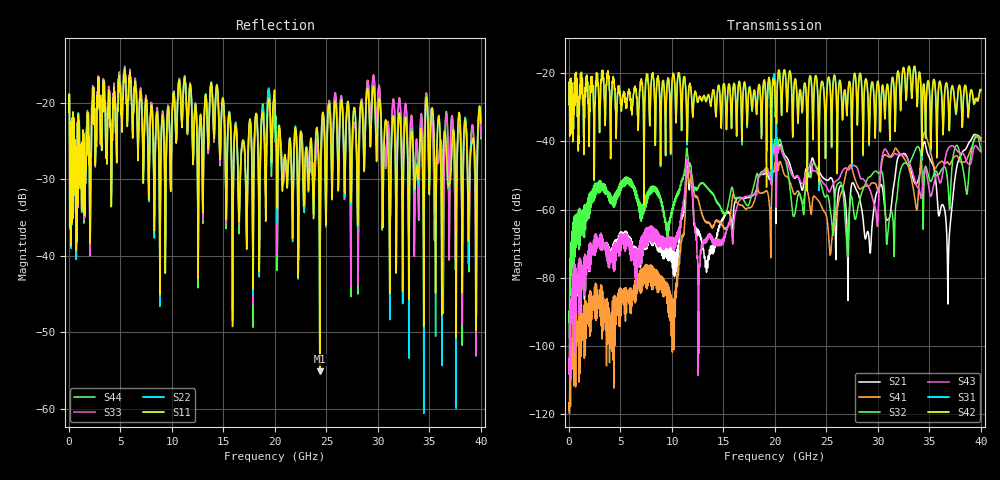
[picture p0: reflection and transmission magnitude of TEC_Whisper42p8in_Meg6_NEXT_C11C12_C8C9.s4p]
! Tyco Electronics Strada Whisper System
! NEXT_C11C12-C8C9
!! SYSTEM DESCRIPTION: Daughtercard-Connector-Backplane-Connector-Daughtercard
!! PCB DESCRIPTION: BP: 250mil, 26 lyrs, Megtron6, bottom layer route, no stub, 6-9-6mil 30" traces; DC: 150mil, 16 lyrs, Megtron6, bottom layer route, no stub, 6-9-6mil 5" traces
!! CONNECTOR DESCRIPTION: STRADA Whisper, Right Angle Receptacle to Vertical Header
!! MODEL DESCRIPTION: Tyco Electronics System 4-port S-parameter
!! MODEL STATUS: Developmental
!! MODEL GEOMETRY: Channel Model
!! MODEL FREQUENCY RANGE: DC to 40 GHz in 10 MHz frequency steps
!! MODEL EDGE RATE LIMITATION: 12.5 ps (Using conservative 0.5/Fmax rule of thumb)
!! TIME-DOMAIN TRANSFORM CAUTIONS:
!! 1.) Do not simulate transient edge rates faster than the number listed above.  Edge rates faster than this number
!!  contain significant spectral content at frequencies above the model's highest frequency.
!! 2.) Even when simulating edge rates that are slower than the number listed above, be aware that the best time
!!  resolution possible with a direct iFFT is (1 / 2Fmax).  As a result, time resolution is typically not adequate
!!  for most time-domain simulations unless tricks such as windowing are used to minimize leakage and aliasing.
!! 3.) Because the model has a uniform frequency step, a direct iFFT will result in an impulse that that has a time
!!  length given by either (1 / Fstep) or (1 / 2Fstep), depending on the transform being used.  Care has been taken
!!  in selecting the frequency step to ensure a settled impulse response for the model.  Therefore, convolution with
!!  the model's impulse response should present no issues.  However, if directly concatenating s-parameter models
!!  in the frequency domain a user must either interpolate necessary interim frequencies or complete impulse response
!!  zero-padding.  Impulse response zero-padding is more difficult, but more accurate.
!! PORT DEFINITIONS:
!! Port  1  ----->  Side A  C8  C11  Side A  <-----  Port  2
!! Port  3  ----->  Side A  C9  C12  Side A  <-----  Port  4
! Created Wed Apr 27 14:05:25 2011
# hz S ma R 50
! 4 Port Network Data from SP1.SP block
! freq  magS11  angS11  magS12  angS12  magS13  angS13  magS14  angS14
!  magS21  angS21  magS22  angS22  magS23  angS23  magS24  angS24
!  magS31  angS31  magS32  angS32  magS33  angS33  magS34  angS34
!  magS41  angS41  magS42  angS42  magS43  angS43  magS44  angS44
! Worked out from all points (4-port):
!   4000 points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, 10 MHz to 40 GHz, reference 50 ohm
!   strongest paths, dB at 10 MHz, 10.01 GHz, 20.01 GHz, 30.01 GHz, 40 GHz:
!     S42: -29.2, -22.5, -27.6, -22.4, -25.0
!     S31: -29.3, -22.6, -23.1, -22.6, -25.3
!     S43: -106.7, -68.7, -41.5, -62.1, -43.1
!     S32: -92.9, -60.1, -39.7, -49.3, -42.8
!     S41: -118.7, -88.7, -46.2, -54.8, -39.8
!     S21: -107.2, -72.1, -41.2, -54.4, -39.1
!   lowest |S11| = -55.1 dB at 24.35 GHz (marker M1), VSWR 1.00, Z = 50 + j0.175 ohm
!   |S11| at or under -10 dB: start of sweep to end of sweep
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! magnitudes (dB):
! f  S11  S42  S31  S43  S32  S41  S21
! 10 MHz  -21.2  -29.2  -29.3  -106.7  -92.9  -118.7  -107.2
! 2.98 GHz  -19.4  -35.7  -35.6  -68.0  -52.5  -83.7  -68.1
! 24.35 GHz  -55.1  -29.5  -29.5  -50.6  -51.2  -58.0  -49.2
! 29.19 GHz  -23.0  -34.1  -34.3  -54.0  -50.4  -53.0  -70.6
! 34.55 GHz  -25.8  -27.6  -27.4  -47.8  -48.3  -37.3  -40.3
! 36.84 GHz  -30.9  -28.9  -28.3  -42.1  -54.4  -46.4  -76.0
! 40 GHz  -22.6  -25.0  -25.3  -43.1  -42.8  -39.8  -39.1
